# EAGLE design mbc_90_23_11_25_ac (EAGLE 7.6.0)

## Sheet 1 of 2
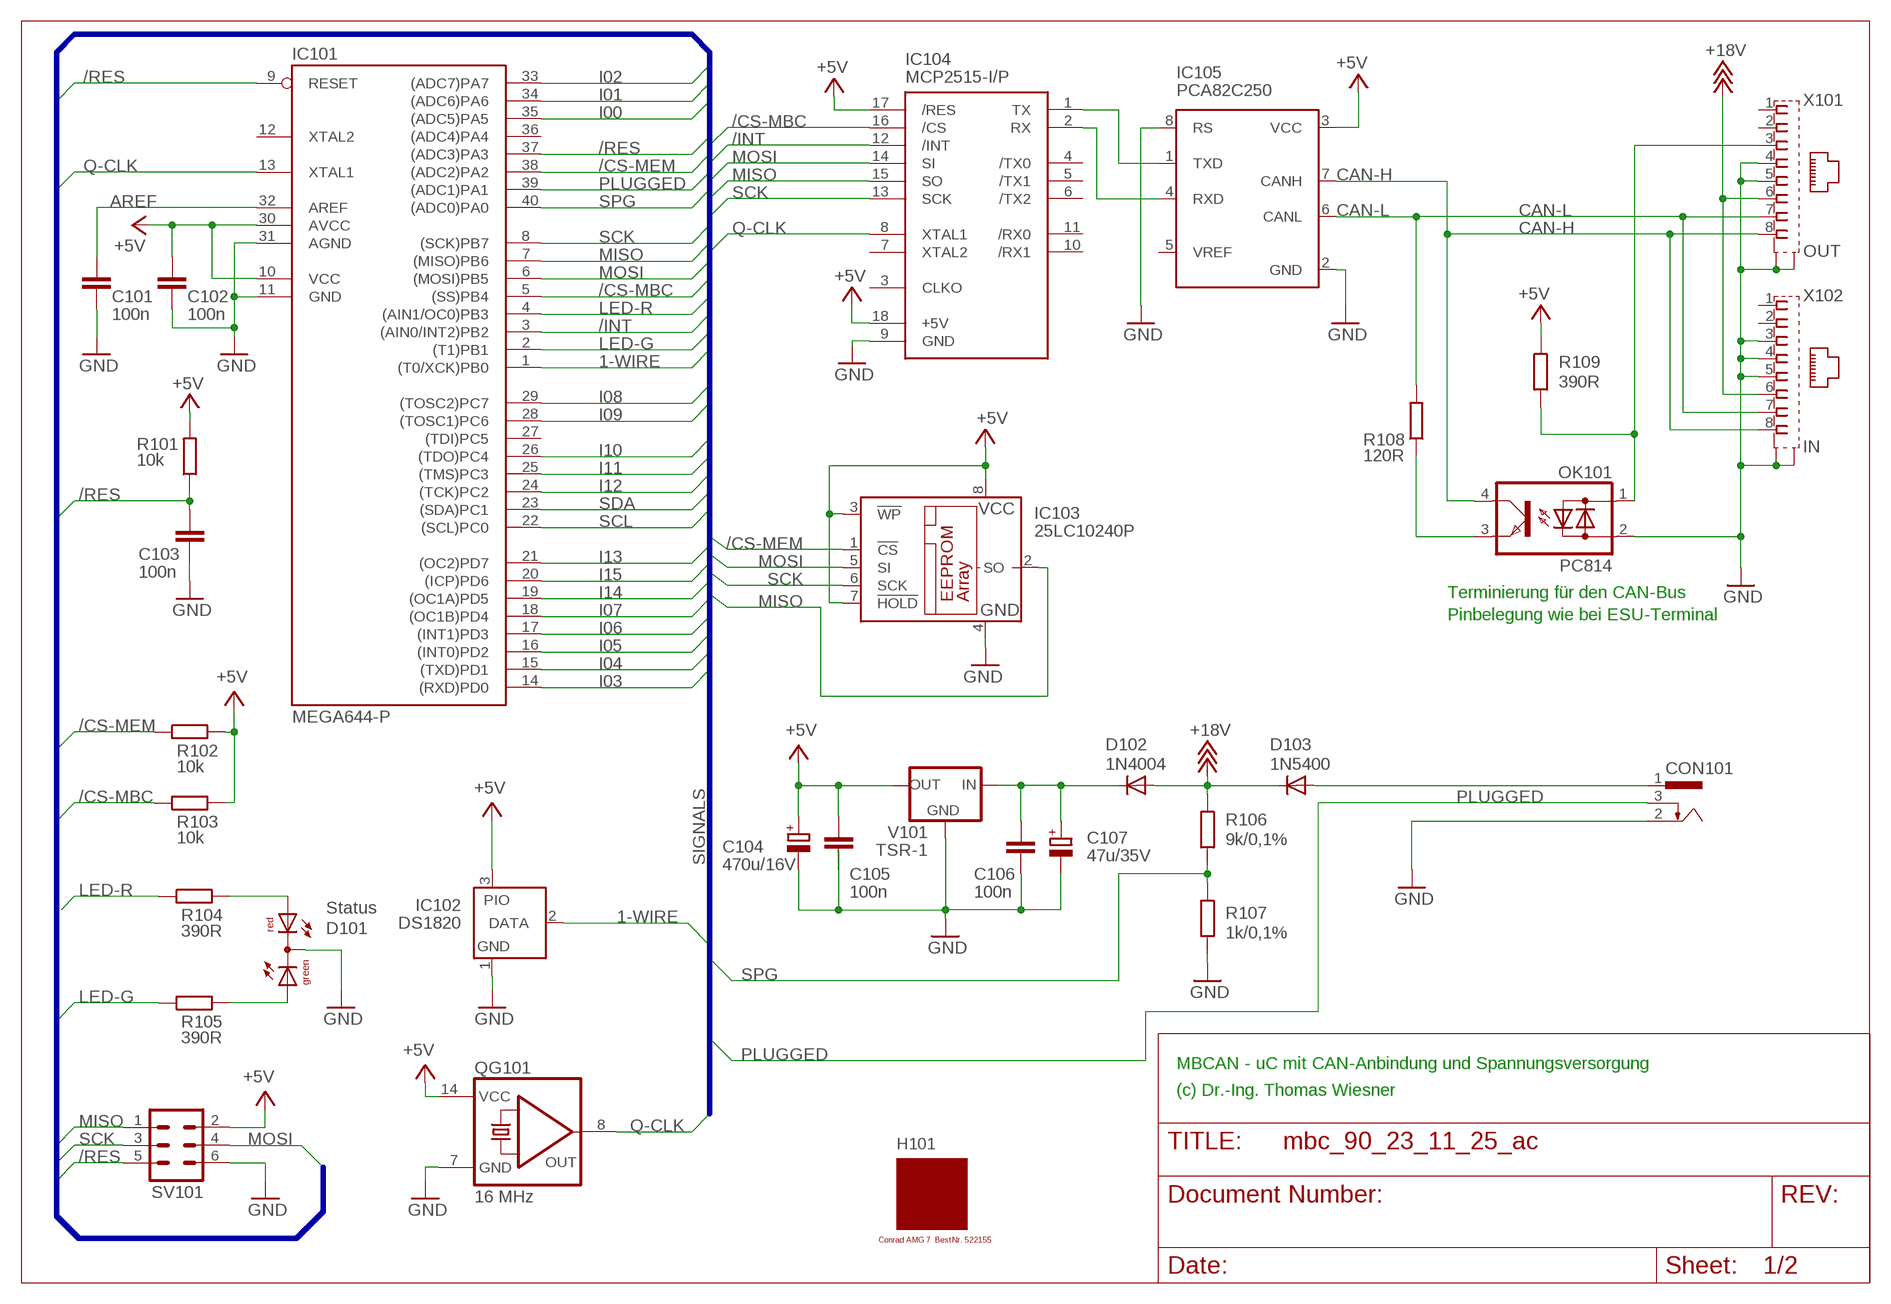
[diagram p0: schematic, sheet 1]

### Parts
C101  100n  C-EU025-025X050  [C025-025X050]
C102  100n  C-EU025-025X050  [C025-025X050]
C103  100n  C-EU025-025X050  [C025-025X050]
C104  470u/16V  CPOL-EUE3.5-8  [E3,5-8]
C105  100n  C-EU025-025X050  [C025-025X050]
C106  100n  C-EU025-025X050  [C025-025X050]
C107  47u/35V  CPOL-EUE2.5-7  [E2,5-7]
CON101  POWER-JACK  [POWER-JACK]
D101  Status  DUOLED5MM  [DUOLED5MM]
D102  1N4004  [DO41-10]
D103  1N5400  [DO201-15]
H101  MODULGEHÄUSE-AMG-7  [MODULGEHÄUSE-1]
IC101  MEGA644-P  MEGA323-P  [DIL40]
IC102  DS1820  DS2405  [TO92-]
IC103  25LC10240P  25LC040P  [DIL8]
IC104  MCP2515-I/P  MCP2510-I/P  [DIL18]
IC105  PCA82C250  [DIL08]
OK101  PC814  [DIL04]
QG101  16 MHz  QG5860  [DIL14S]
R101  10k  R-EU_0207/10  [0207/10]
R102  10k  R-EU_0207/10  [0207/10]
R103  10k  R-EU_0207/10  [0207/10]
R104  390R  R-EU_0207/10  [0207/10]
R105  390R  R-EU_0207/10  [0207/10]
R106  9k/0,1%  R-EU_0207/10  [0207/10]
R107  1k/0,1%  R-EU_0207/10  [0207/10]
R108  120R  R-EU_0207/10  [0207/10]
R109  390R  R-EU_0207/10  [0207/10]
SV101  ML6  [ML6]
V101  TSR-1  [TRACO-TSR-1]
X101  OUT  0446200002  [0446200002]
X102  IN  0446200002  [0446200002]

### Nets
1-WIRE: IC101.1((T0/XCK)PB0) IC102.2(DATA)
+5V: C102.1 C104.+ C105.1 IC101.10(VCC) IC101.30(AVCC) IC102.3(PIO) IC103.3(!WP) IC103.7(!HOLD) IC103.8(VCC) IC104.17(/RES) IC104.18(+5V) IC105.3(VCC) QG101.14(VCC) R101.2 R102.2 R103.2 R109.1 SV101.2 V101.OUT ; also sheet 2
+18V: D102.A D103.C R106.1 X101.6 X102.6
/CS-MBC: IC101.5((SS)PB4) IC104.16(/CS) R103.1
/CS-MEM: IC101.38((ADC2)PA2) IC103.1(!CS) R102.1
/INT: IC101.3((AIN0/INT2)PB2) IC104.12(/INT)
/RES: C103.1 IC101.9(RESET) IC101.37((ADC3)PA3) R101.1 SV101.5
AREF: C101.1 IC101.32(AREF)
CAN-H: IC105.7(CANH) OK101.4(C) X101.8 X102.8
CAN-L: IC105.6(CANL) R108.2 X101.7 X102.7
GND: C101.2 C102.2 C103.2 C104.- C105.2 C106.2 C107.- CON101.2 D101.K(C) IC101.11(GND) IC101.31(AGND) IC102.1(GND) IC103.4(GND) IC104.9(GND) IC105.2(GND) IC105.8(RS) QG101.7(GND) R107.2 SV101.6 V101.GND X101.4 X101.5 X101.S@1(S1) X101.S@2(S2) X102.3 X102.4 X102.5 X102.S@1(S1) X102.S@2(S2) ; also sheet 2
I00: IC101.35((ADC5)PA5) ; also sheet 2
I01: IC101.34((ADC6)PA6) ; also sheet 2
I02: IC101.33((ADC7)PA7) ; also sheet 2
I03: IC101.14((RXD)PD0) ; also sheet 2
I04: IC101.15((TXD)PD1) ; also sheet 2
I05: IC101.16((INT0)PD2) ; also sheet 2
I06: IC101.17((INT1)PD3) ; also sheet 2
I07: IC101.18((OC1B)PD4) ; also sheet 2
I08: IC101.29((TOSC2)PC7) ; also sheet 2
I09: IC101.28((TOSC1)PC6) ; also sheet 2
I10: IC101.26((TDO)PC4) ; also sheet 2
I11: IC101.25((TMS)PC3) ; also sheet 2
I12: IC101.24((TCK)PC2) ; also sheet 2
I13: IC101.21((OC2)PD7) ; also sheet 2
I14: IC101.19((OC1A)PD5) ; also sheet 2
I15: IC101.20((ICP)PD6) ; also sheet 2
LED-G: IC101.2((T1)PB1) R105.1
LED-R: IC101.4((AIN1/OC0)PB3) R104.1
MISO: IC101.7((MISO)PB6) IC103.2(SO) IC104.15(SO) SV101.1
MOSI: IC101.6((MOSI)PB5) IC103.5(SI) IC104.14(SI) SV101.4
N$1: IC104.1(TX) IC105.1(TXD)
N$2: IC104.2(RX) IC105.4(RXD)
N$4: OK101.3(E) R108.1
N$6: C106.1 C107.+ D102.C V101.IN
N$7: OK101.1(AC1) R109.2 X101.3
N$9: D101.AR R104.2
N$13: D101.AG R105.2
PLUGGED: CON101.3 IC101.39((ADC1)PA1)
Q-CLK: IC101.13(XTAL1) IC104.8(XTAL1) QG101.8(OUT)
SCK: IC101.8((SCK)PB7) IC103.6(SCK) IC104.13(SCK) SV101.3
SCL: IC101.22((SCL)PC0) ; also sheet 2
SDA: IC101.23((SDA)PC1) ; also sheet 2
SPG: IC101.40((ADC0)PA0) R106.2 R107.1
V-NETZTEIL1: CON101.1 D103.A
Unconnected: IC101.12(XTAL2) IC101.27((TDI)PC5) IC101.36((ADC4)PA4) IC104.3(CLKO) IC104.4(/TX0) IC104.5(/TX1) IC104.6(/TX2) IC104.7(XTAL2) IC104.10(/RX1) IC104.11(/RX0) IC105.5(VREF) OK101.2(AC2) X101.1 X101.2 X102.1 X102.2

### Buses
SIGNALS

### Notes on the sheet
- Terminierung für den CAN-Bus
- Pinbelegung wie bei ESU-Terminal
- MBCAN - uC mit CAN-Anbindung und Spannungsversorgung
- (c) Dr.-Ing. Thomas Wiesner

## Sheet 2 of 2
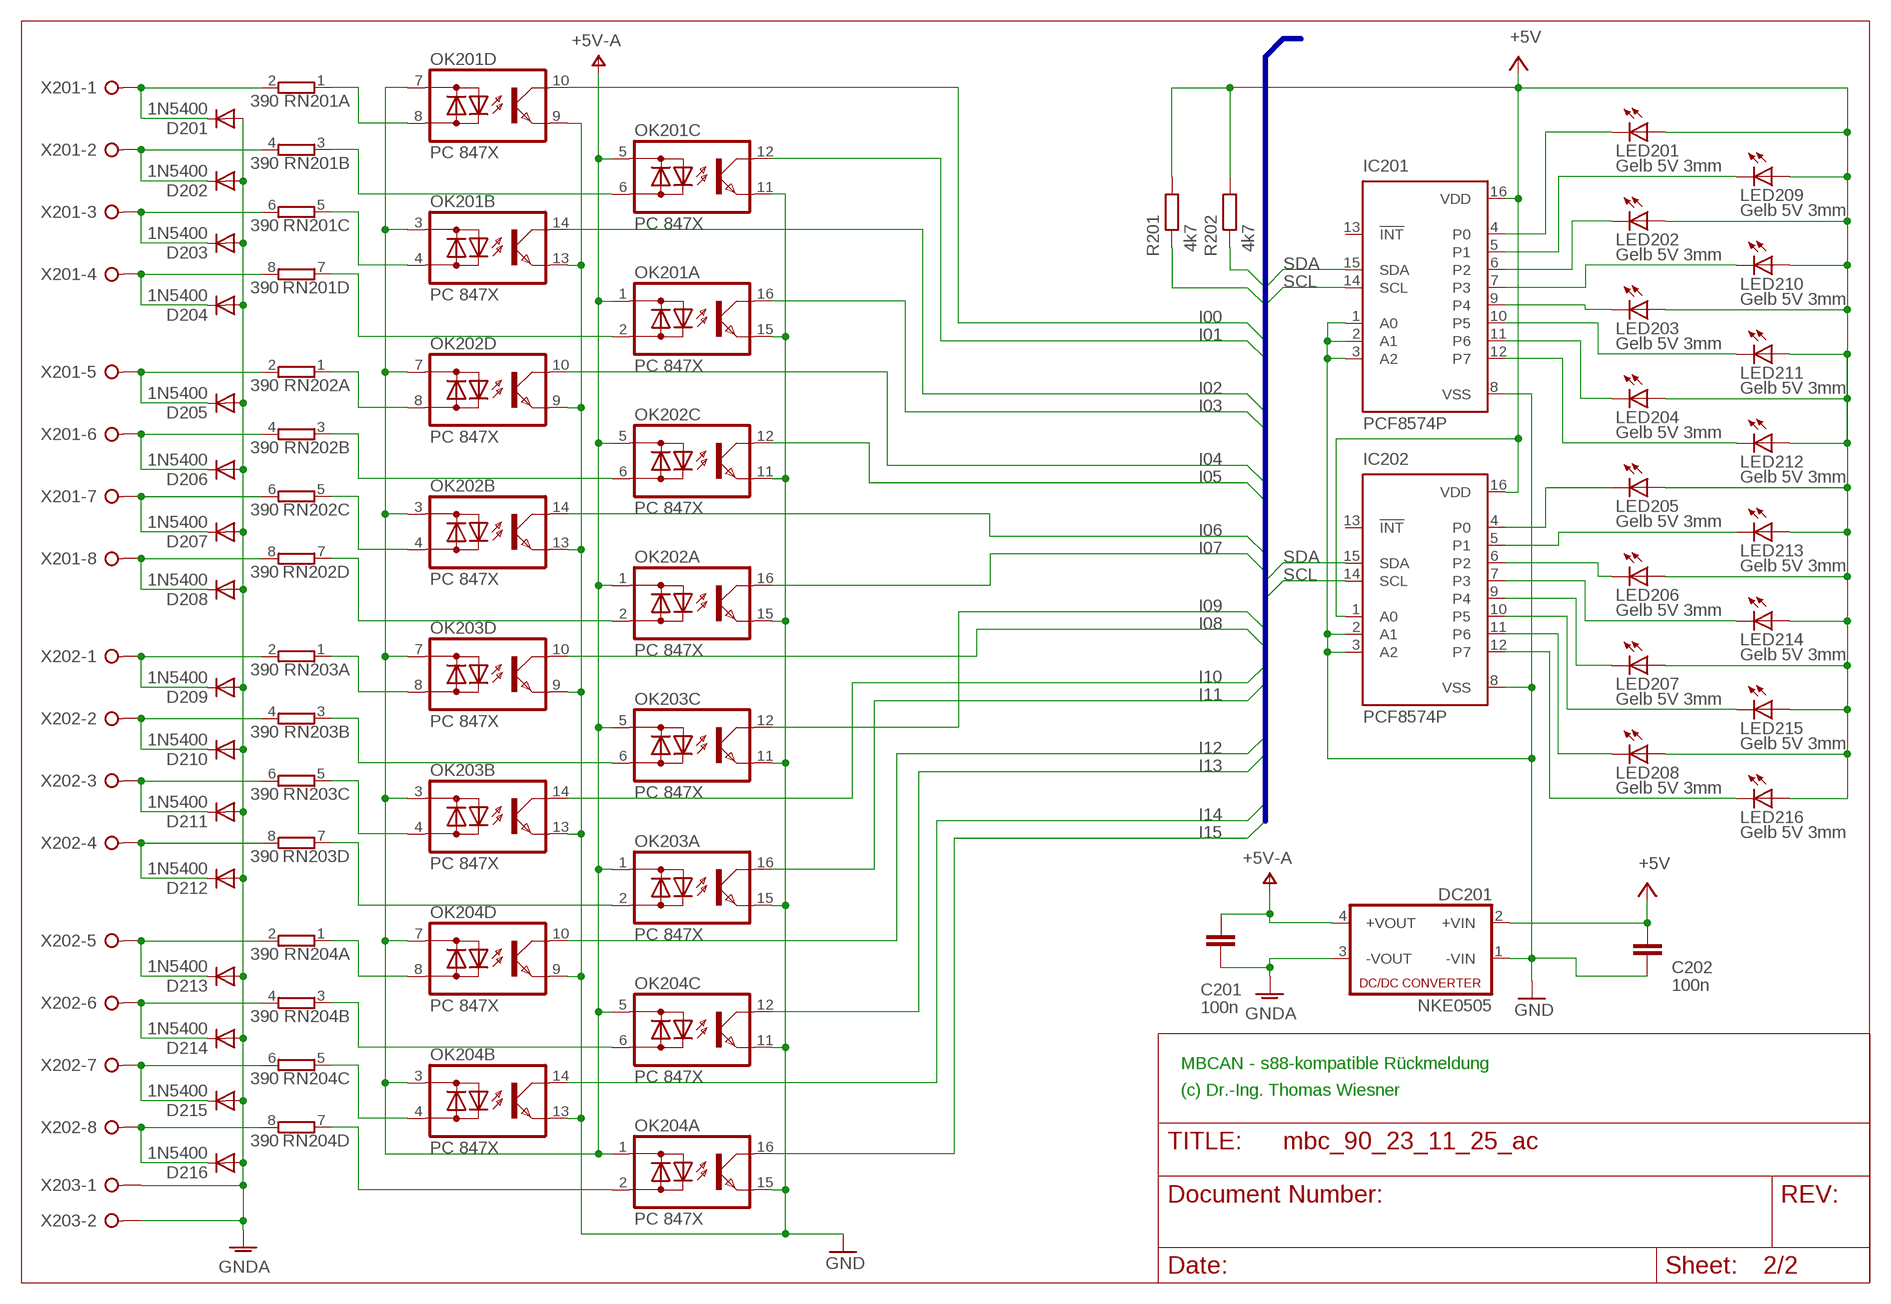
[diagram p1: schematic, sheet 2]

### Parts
C201  100n  C-EU025-025X050  [C025-025X050]
C202  100n  C-EU025-025X050  [C025-025X050]
D201  1N5400  [DO201-15]
D202  1N5400  [DO201-15]
D203  1N5400  [DO201-15]
D204  1N5400  [DO201-15]
D205  1N5400  [DO201-15]
D206  1N5400  [DO201-15]
D207  1N5400  [DO201-15]
D208  1N5400  [DO201-15]
D209  1N5400  [DO201-15]
D210  1N5400  [DO201-15]
D211  1N5400  [DO201-15]
D212  1N5400  [DO201-15]
D213  1N5400  [DO201-15]
D214  1N5400  [DO201-15]
D215  1N5400  [DO201-15]
D216  1N5400  [DO201-15]
DC201  NKE0505  NME  [NME]
IC201  PCF8574P  [DIL16]
IC202  PCF8574P  [DIL16]
LED201  Gelb 5V 3mm  LED3MM  [LED3MM]
LED202  Gelb 5V 3mm  LED3MM  [LED3MM]
LED203  Gelb 5V 3mm  LED3MM  [LED3MM]
LED204  Gelb 5V 3mm  LED3MM  [LED3MM]
LED205  Gelb 5V 3mm  LED3MM  [LED3MM]
LED206  Gelb 5V 3mm  LED3MM  [LED3MM]
LED207  Gelb 5V 3mm  LED3MM  [LED3MM]
LED208  Gelb 5V 3mm  LED3MM  [LED3MM]
LED209  Gelb 5V 3mm  LED3MM  [LED3MM]
LED210  Gelb 5V 3mm  LED3MM  [LED3MM]
LED211  Gelb 5V 3mm  LED3MM  [LED3MM]
LED212  Gelb 5V 3mm  LED3MM  [LED3MM]
LED213  Gelb 5V 3mm  LED3MM  [LED3MM]
LED214  Gelb 5V 3mm  LED3MM  [LED3MM]
LED215  Gelb 5V 3mm  LED3MM  [LED3MM]
LED216  Gelb 5V 3mm  LED3MM  [LED3MM]
OK201  PC 847X  TIL196  [DIL16]
OK202  PC 847X  TIL196  [DIL16]
OK203  PC 847X  TIL196  [DIL16]
OK204  PC 847X  TIL196  [DIL16]
R201  4k7  R-EU_0207/10  [0207/10]
R202  4k7  R-EU_0207/10  [0207/10]
RN201  390  E4R  [SIL8]
RN202  390  E4R  [SIL8]
RN203  390  E4R  [SIL8]
RN204  390  E4R  [SIL8]
X201  W237-08P  [W237-8P]
X202  W237-08P  [W237-8P]
X203  W237-02P  [W237-132]

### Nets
+5V: C202.1 DC201.2(+VIN) IC201.16(VDD) IC202.1(A0) IC202.16(VDD) LED201.A LED202.A LED203.A LED204.A LED205.A LED206.A LED207.A LED208.A LED209.A LED210.A LED211.A LED212.A LED213.A LED214.A LED215.A LED216.A R201.2 R202.2 ; also sheet 1
GND: C202.2 DC201.1(-VIN) IC201.1(A0) IC201.2(A1) IC201.3(A2) IC201.8(VSS) IC202.2(A1) IC202.3(A2) IC202.8(VSS) OK201.9(D:E) OK201.11(C:E) OK201.13(B:E) OK201.15(A:E) OK202.9(D:E) OK202.11(C:E) OK202.13(B:E) OK202.15(A:E) OK203.9(D:E) OK203.11(C:E) OK203.13(B:E) OK203.15(A:E) OK204.9(D:E) OK204.11(C:E) OK204.13(B:E) OK204.15(A:E) ; also sheet 1
GNDA: C201.2 D201.A D202.A D203.A D204.A D205.A D206.A D207.A D208.A D209.A D210.A D211.A D212.A D213.A D214.A D215.A D216.A DC201.3(-VOUT) X203.1 X203.2
I00: OK201.10(D:C) ; also sheet 1
I01: OK201.12(C:C) ; also sheet 1
I02: OK201.14(B:C) ; also sheet 1
I03: OK201.16(A:C) ; also sheet 1
I04: OK202.10(D:C) ; also sheet 1
I05: OK202.12(C:C) ; also sheet 1
I06: OK202.14(B:C) ; also sheet 1
I07: OK202.16(A:C) ; also sheet 1
I08: OK203.10(D:C) ; also sheet 1
I09: OK203.12(C:C) ; also sheet 1
I10: OK203.14(B:C) ; also sheet 1
I11: OK203.16(A:C) ; also sheet 1
I12: OK204.10(D:C) ; also sheet 1
I13: OK204.12(C:C) ; also sheet 1
I14: OK204.14(B:C) ; also sheet 1
I15: OK204.16(A:C) ; also sheet 1
N$15: IC201.9(P4) LED203.K(C)
N$16: D215.C RN204.6 X202.7
N$17: D216.C RN204.8 X202.8
N$18: D213.C RN204.2 X202.5
N$19: D214.C RN204.4 X202.6
N$20: D211.C RN203.6 X202.3
N$21: D212.C RN203.8 X202.4
N$22: D209.C RN203.2 X202.1
N$23: D210.C RN203.4 X202.2
N$24: D207.C RN202.6 X201.7
N$25: D208.C RN202.8 X201.8
N$26: D205.C RN202.2 X201.5
N$27: D206.C RN202.4 X201.6
N$28: D203.C RN201.6 X201.3
N$29: D204.C RN201.8 X201.4
N$30: D201.C RN201.2 X201.1
N$31: IC201.10(P5) LED211.K(C)
N$32: OK204.2(A:AC2) RN204.7
N$35: OK204.4(B:AC2) RN204.5
N$36: OK204.6(C:AC2) RN204.3
N$37: OK204.8(D:AC2) RN204.1
N$38: OK203.2(A:AC2) RN203.7
N$39: OK203.4(B:AC2) RN203.5
N$40: OK203.6(C:AC2) RN203.3
N$41: OK203.8(D:AC2) RN203.1
N$42: OK202.2(A:AC2) RN202.7
N$43: OK202.4(B:AC2) RN202.5
N$44: OK202.6(C:AC2) RN202.3
N$45: OK202.8(D:AC2) RN202.1
N$46: OK201.2(A:AC2) RN201.7
N$47: D202.C RN201.4 X201.2
N$48: OK201.4(B:AC2) RN201.5
N$49: IC202.4(P0) LED205.K(C)
N$50: IC201.4(P0) LED201.K(C)
N$51: IC201.5(P1) LED209.K(C)
N$52: IC201.6(P2) LED202.K(C)
N$53: IC201.7(P3) LED210.K(C)
N$54: IC201.11(P6) LED204.K(C)
N$55: IC201.12(P7) LED212.K(C)
N$56: IC202.9(P4) LED207.K(C)
N$57: IC202.5(P1) LED213.K(C)
N$58: IC202.6(P2) LED206.K(C)
N$59: IC202.7(P3) LED214.K(C)
N$60: IC202.10(P5) LED215.K(C)
N$61: IC202.11(P6) LED208.K(C)
N$62: IC202.12(P7) LED216.K(C)
N$64: OK201.6(C:AC2) RN201.3
N$65: OK201.8(D:AC2) RN201.1
SCL: IC201.14(SCL) IC202.14(SCL) R201.1 ; also sheet 1
SDA: IC201.15(SDA) IC202.15(SDA) R202.1 ; also sheet 1
V+: C201.1 DC201.4(+VOUT) OK201.1(A:AC1) OK201.3(B:AC1) OK201.5(C:AC1) OK201.7(D:AC1) OK202.1(A:AC1) OK202.3(B:AC1) OK202.5(C:AC1) OK202.7(D:AC1) OK203.1(A:AC1) OK203.3(B:AC1) OK203.5(C:AC1) OK203.7(D:AC1) OK204.1(A:AC1) OK204.3(B:AC1) OK204.5(C:AC1) OK204.7(D:AC1) ; supply symbol labelled +5V-A
Unconnected: IC201.13(!INT) IC202.13(!INT)

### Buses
B$1

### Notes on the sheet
- MBCAN - s88-kompatible Rückmeldung
- (c) Dr.-Ing. Thomas Wiesner

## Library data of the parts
C101-C103 C105 C106 C201 C202 = rcl:C-EU: CAPACITOR, European symbol
C104 C107 = rcl:CPOL-EU: POLARIZED CAPACITOR, European symbol
CON101 = mbc:POWER-JACK: Power-Stecker für 2,5 mm Hohlbuchse
D101 = led:DUOLED5MM: DUO LED 2 colors, 5 mm, round
D102 = diode:1N4004: DIODE
D103 D201-D216 = diode:1N5400: DIODE
DC201 = dc-dc-converter:NME: DC-DC CONVERTER; MF: C & D TECHNOLOGIES, INC; MPN: NME1205D; OC_FARNELL: 1021466; OC_NEWARK: 98B8198
H101 = mbc:MODULGEHÄUSE-AMG-7: Gehäuse
IC101 = atmel:MEGA323-P: MICROCONTROLLER 32 Kbytes FLASH 2 Kbytes SRAM 1 Kbytes EEPROM USART 8-channel 10 bit ADC Source: avr.lbr; OC_FARNELL: unknown; OC_NEWARK: unknown
IC102 = maxim:DS2405: Addressable Switch DALLAS Semiconductor; MF: DALLAS SEMICONDUCTOR; MPN: DS2405; OC_FARNELL: 1188025; OC_NEWARK: 06F4645
IC103 = microchip:25*: Serial EEPROM 4K/ 8K , SPI bus; MF: MICROCHIP; MPN: 25LC040/P; OC_FARNELL: 9758100; OC_NEWARK: 96K4091
IC104 = mbc:MCP2510: BASIC-CAN 2.0a Controller Stand-alone CAN controller von Microchip
IC105 = micro-philips:PCA82C250: CAN CONTROLLER INTERFACE; OC_FARNELL: 3692358; OC_NEWARK: unknown
IC201 IC202 = micro-philips:PCF8574: I2C-Bus Remote 8-bit I/O expander http://www.semiconductors.philips.com/acrobat_download/datasheets/PCF8574_4.pdf; MPN: PCF8574PN; OC_FARNELL: 204020; OC_NEWARK: 11N8515
LED201-LED216 = led:LED: LED
OK101 = optocoupler:PC814: SHARP OPTO COUPLER; OC_FARNELL: 9707662; OC_NEWARK: unknown
OK201-OK204 = optocoupler:TIL196: TEXAS INSTRUMENTS OPTO COUPLER; MPN: TIL 196; OC_FARNELL: 1683367; OC_NEWARK: 05R6476
QG101 = crystal:QG5860: CRYSTAL RESONATOR; OC_FARNELL: unknown; OC_NEWARK: unknown
R101-R109 R201 R202 = resistor:R-EU_: RESISTOR, European symbol
RN201-RN204 = resistor-sil:E4R: SIL RESISTOR; OC_FARNELL: unknown; OC_NEWARK: unknown
SV101 = con-ml:ML6: HARTING; OC_FARNELL: unknown; OC_NEWARK: unknown
V101 = mbc:TSR-1: Spannungsregler Hersteller: TRACO Typ: TSR-1 5V: TSR 1-2450 Spg: 5V Strom: 1A Reichelt TSR 1-2450
X101 X102 = mbc:0446200002: RJ-45 INVERTED MODULAR JACK ASSEMBLY WITH RJ-11 KEEPOUT FEATURE Source: Data sheet MOLEX 0446200002 BUCHSE, RJ45, GESCHIRMT Source: Farnell; MF: MOLEX; MPN: 0446200002; OC_FARNELL: 9251910
X201 X202 = con-wago-508:W237-08P: WAGO SREW CLAMP; OC_FARNELL: unknown; OC_NEWARK: unknown
X203 = con-wago-508:W237-02P: WAGO SREW CLAMP; OC_FARNELL: unknown; OC_NEWARK: unknown

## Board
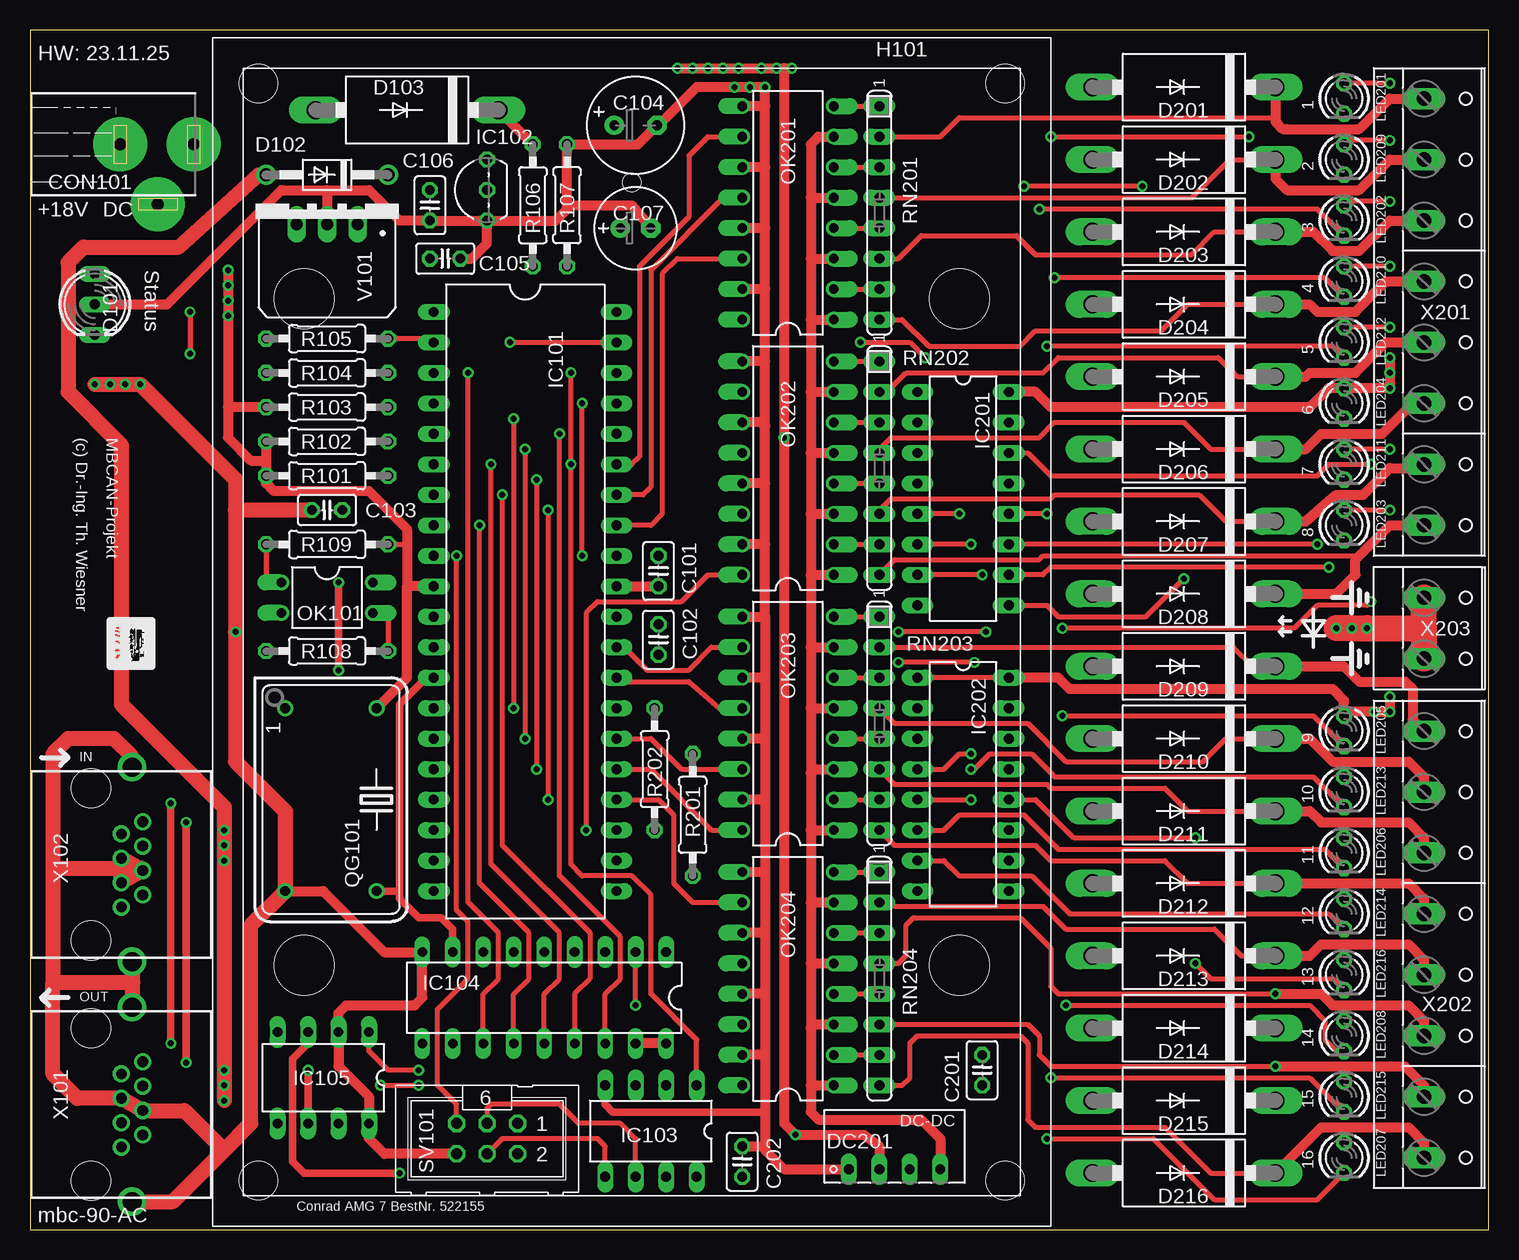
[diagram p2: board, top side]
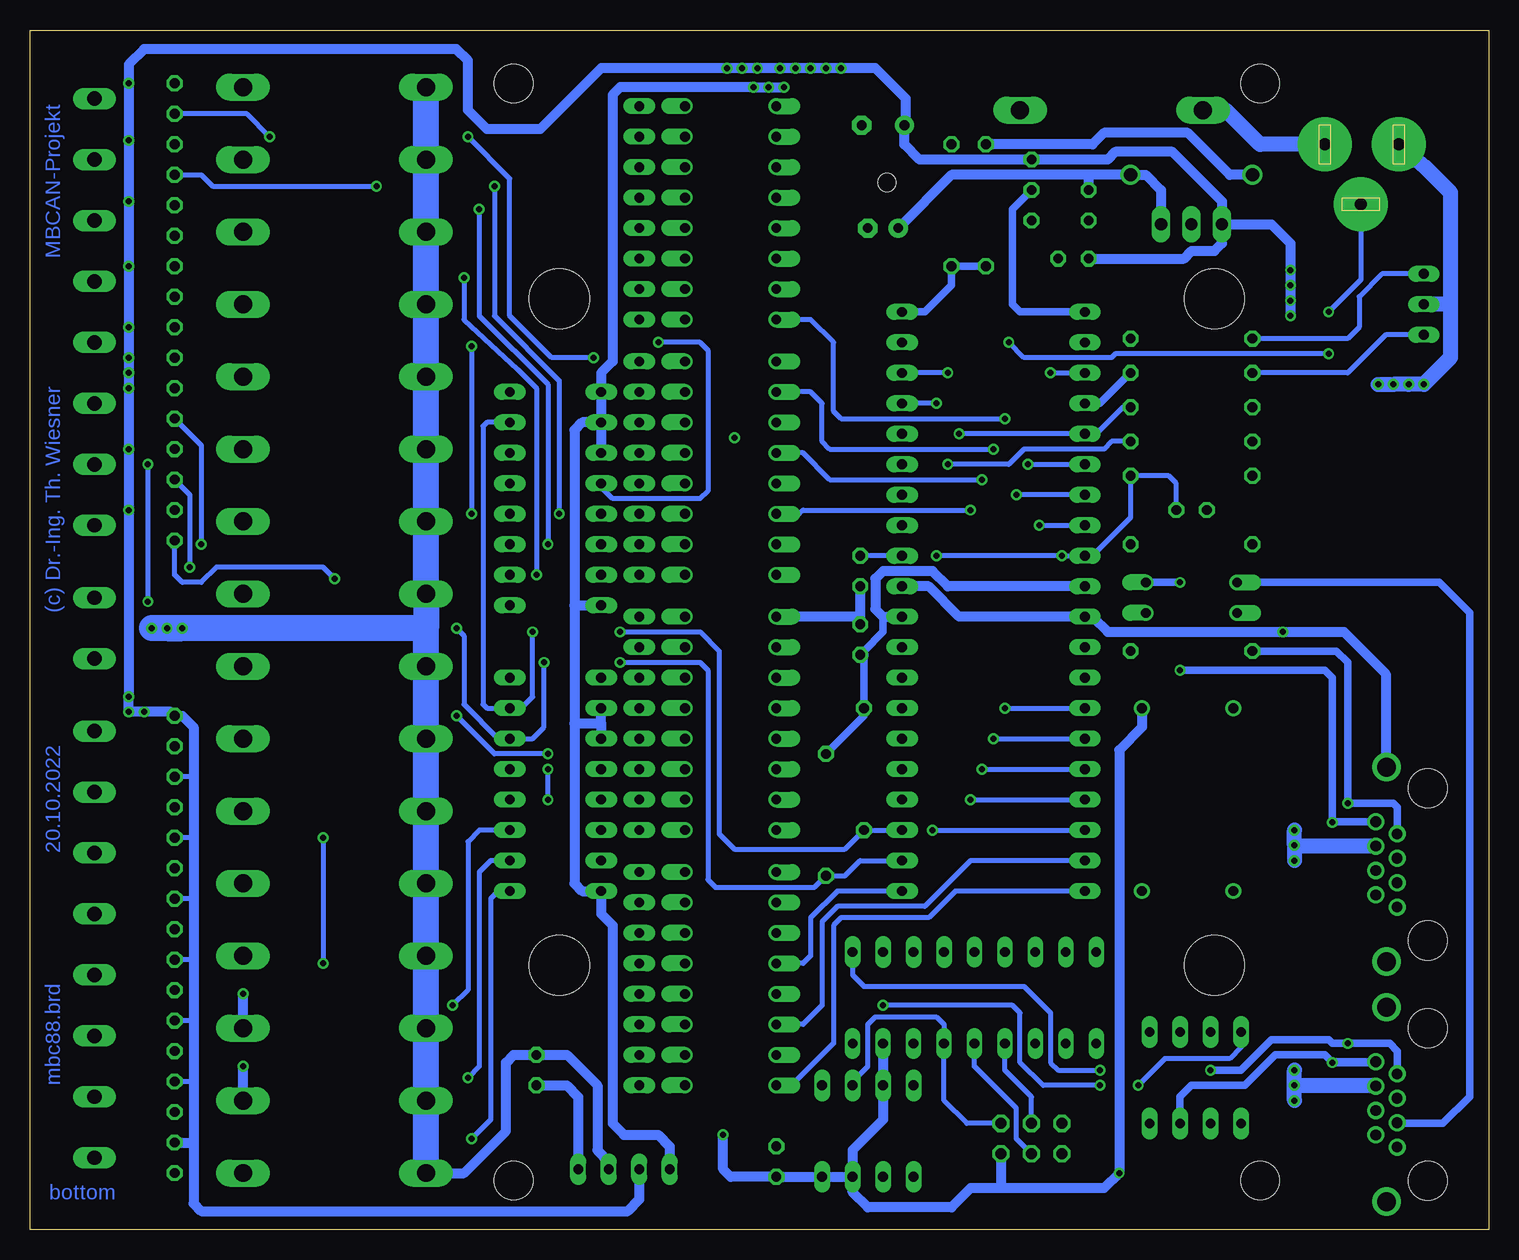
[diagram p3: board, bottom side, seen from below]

Size 121.59 x 99.99 mm. Coordinates in mm from the lower left corner, seen from the top.
Outline: 0,99.99 0,0 121.59,0 121.59,99.99 0,99.99
Copper layers (1*16): Top 0.035mm / dielectric 1.5mm / Bottom 0.035mm
Design rules "default *": minimum track width 10mil, minimum drill 0.5mm, track to track 8mil, track to pad 8mil, pad to pad 8mil, via to via 8mil, smd to smd 8mil, copper to edge 40mil, drill to drill 8mil, minimum pad ring 10mil, minimum via ring 8mil, stop-mask expansion 4mil, vias tented up to drill 0mil, thermal gap 10mil

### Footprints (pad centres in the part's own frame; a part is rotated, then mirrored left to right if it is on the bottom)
C025-025X050 = drill 0.813 octagon: 1 -1.27,0; 2 1.27,0
E3,5-8 = drill 0.813 pad 1.6: + -1.778,0 | drill 0.813 pad 1.6 octagon: - 1.778,0
E2,5-7 = drill 0.813 pad 1.6: + -1.27,0 | drill 0.813 pad 1.6 octagon: - 1.27,0
POWER-JACK = drill 1 pad 4.5: 1 0,6.03; 2 0,-0.12; 3 5,3.03
DUOLED5MM = drill 0.813 long: AG -2.54,0; AR 2.54,0; K 0,0
DO41-10 = drill 1.118: A 5.08,0; C -5.08,0
DO201-15 = drill 1.499 long: A 7.62,0; C -7.62,0
NME = drill 0.813 long: 1 0,3.81; 2 0,1.27; 3 0,-1.27; 4 0,-3.81
MODULGEHÄUSE-1 = hole 3.2: -45.72,-31.115; -45.72,31.115; 45.72,31.115; 45.72,-31.115 | hole 5: -27.781,-27.305; 27.781,-27.305; -27.781,27.305; 27.781,27.305 | hole 1.5: -37.465,0
DIL40 = drill 0.813 long: 1 -24.13,-7.62; 2 -21.59,-7.62; 3 -19.05,-7.62; 4 -16.51,-7.62; 5 -13.97,-7.62; 6 -11.43,-7.62; 7 -8.89,-7.62; 8 -6.35,-7.62; 9 -3.81,-7.62; 10 -1.27,-7.62; 11 1.27,-7.62; 12 3.81,-7.62; 13 6.35,-7.62; 14 8.89,-7.62; 15 11.43,-7.62; 16 13.97,-7.62; 17 16.51,-7.62; 18 19.05,-7.62; 19 21.59,-7.62; 20 24.13,-7.62; 21 24.13,7.62; 22 21.59,7.62; 23 19.05,7.62; 24 16.51,7.62; 25 13.97,7.62; 26 11.43,7.62; 27 8.89,7.62; 28 6.35,7.62; 29 3.81,7.62; 30 1.27,7.62; 31 -1.27,7.62; 32 -3.81,7.62; 33 -6.35,7.62; 34 -8.89,7.62; 35 -11.43,7.62; 36 -13.97,7.62; 37 -16.51,7.62; 38 -19.05,7.62; 39 -21.59,7.62; 40 -24.13,7.62
TO92- = drill 0.813 octagon: 1 -2.54,0; 2 0,0; 3 2.54,0
DIL8 = drill 0.813 long: 1 -3.81,-3.81; 2 -1.27,-3.81; 3 1.27,-3.81; 4 3.81,-3.81; 5 3.81,3.81; 6 1.27,3.81; 7 -1.27,3.81; 8 -3.81,3.81
DIL18 = drill 0.813 long: 1 -10.16,-3.81; 2 -7.62,-3.81; 3 -5.08,-3.81; 4 -2.54,-3.81 | drill 0.8 long: 5 0,-3.81; 6 2.54,-3.81; 7 5.08,-3.81; 8 7.62,-3.81; 9 10.16,-3.81; 10 10.16,3.81; 11 7.62,3.81; 12 5.08,3.81; 13 2.54,3.81; 14 0,3.81; 15 -2.54,3.81; 16 -5.08,3.81; 17 -7.62,3.81; 18 -10.16,3.81
DIL08 = drill 0.813 long: 1 -3.81,-3.81; 2 -1.27,-3.81; 3 1.27,-3.81; 4 3.81,-3.81; 5 3.81,3.81; 6 1.27,3.81; 7 -1.27,3.81; 8 -3.81,3.81
DIL16 = drill 0.813 long: 1 -8.89,-3.81; 2 -6.35,-3.81; 3 -3.81,-3.81; 4 -1.27,-3.81; 5 1.27,-3.81; 6 3.81,-3.81; 7 6.35,-3.81; 8 8.89,-3.81; 9 8.89,3.81; 10 6.35,3.81; 11 3.81,3.81; 12 1.27,3.81; 13 -1.27,3.81; 14 -3.81,3.81; 15 -6.35,3.81; 16 -8.89,3.81
LED3MM = drill 0.813 octagon: A -1.27,0; K 1.27,0
DIL04 = drill 0.813 offset: 1 -1.27,-3.81; 2 1.27,-3.81; 3 1.27,3.81; 4 -1.27,3.81
DIL16' = drill 0.813 offset: 1 -8.89,-3.81; 2 -6.35,-3.81; 3 -3.81,-3.81; 4 -1.27,-3.81; 5 1.27,-3.81; 6 3.81,-3.81; 7 6.35,-3.81; 8 8.89,-3.81; 9 8.89,3.81; 10 6.35,3.81; 11 3.81,3.81; 12 1.27,3.81; 13 -1.27,3.81; 14 -3.81,3.81; 15 -6.35,3.81; 16 -8.89,3.81
DIL14S = drill 0.813: 1 -7.62,-3.81; 7 7.62,-3.81; 8 7.62,3.81; 14 -7.62,3.81
0207/10 = drill 0.813 octagon: 1 -5.08,0; 2 5.08,0
SIL8 = drill 0.813 long: 1 -8.89,0; 2 -6.35,0; 3 -3.81,0; 4 -1.27,0; 5 1.27,0; 6 3.81,0; 7 6.35,0; 8 8.89,0
ML6 = drill 0.914 octagon: 1 -2.54,-1.27; 2 -2.54,1.27; 3 0,-1.27; 4 0,1.27; 5 2.54,-1.27; 6 2.54,1.27
TRACO-TSR-1 = drill 1.016 long: GND 0,2.54; IN -2.54,2.54; OUT 2.54,2.54
0446200002 = drill 0.889 pad 1.422: 1 3.556,2.54; 2 2.54,4.318; 3 1.524,2.54; 4 0.508,4.318; 5 -0.508,2.54; 6 -1.524,4.318; 7 -2.54,2.54; 8 -3.556,4.318 | drill 1.575 pad 2.286: S@1 -8.103,3.429; S@2 8.103,3.429 | hole 3.251: 6.35,0; -6.35,0
W237-8P = drill 1.194 long: 1 -17.78,-0.635; 2 -12.7,-0.635; 3 -7.62,-0.635; 4 -2.54,-0.635; 5 2.54,-0.635; 6 7.62,-0.635; 7 12.7,-0.635; 8 17.78,-0.635
W237-132 = drill 1.194 long: 1 -2.54,-0.635; 2 2.54,-0.635

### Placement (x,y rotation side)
C101  52.39,54.91 270 top
C102  52.39,49.19 90 top
C103  24.77,59.99 180 top
C104  50.48,92.06 0 top
C105  34.61,80.94 0 top
C106  33.34,85.39 270 top
C107  50.48,83.48 0 top
C201  79.38,13.32 90 top
C202  59.37,5.7 90 top
CON101  7.62,90.47 270 top
D101  5.4,77.13 270 top
D102  24.77,87.93 180 top
D103  31.43,93.33 180 top
D201  96.2,95.23 180 top
D202  96.2,89.2 180 top
D203  96.2,83.17 180 top
D204  96.2,77.13 180 top
D205  96.2,71.1 180 top
D206  96.2,65.07 180 top
D207  96.2,59.03 180 top
D208  96.2,53 180 top
D209  96.2,46.97 180 top
D210  96.2,40.94 180 top
D211  96.2,34.9 180 top
D212  96.2,28.87 180 top
D213  96.2,22.84 180 top
D214  96.2,16.81 180 top
D215  96.2,10.78 180 top
D216  96.2,4.74 180 top
DC201  72.07,5.06 90 top
H101  50.16,49.83 270 top
IC101  41.27,52.37 270 top
IC102  38.1,86.66 90 top
IC103  51.75,8.24 180 top
IC104  42.86,19.35 180 top
IC105  24.45,12.68 180 top
IC201  77.79,60.94 270 top
IC202  77.79,37.13 270 top
LED201  109.54,94.28 270 top
LED202  109.54,84.12 270 top
LED203  109.54,58.72 270 top
LED204  109.54,68.88 270 top
LED205  109.54,41.57 270 top
LED206  109.54,31.41 270 top
LED207  109.54,6.01 270 top
LED208  109.54,16.17 270 top
LED209  109.54,89.2 270 top
LED210  109.54,79.04 270 top
LED211  109.54,63.8 270 top
LED212  109.54,73.96 270 top
LED213  109.54,36.49 270 top
LED214  109.54,26.33 270 top
LED215  109.54,11.09 270 top
LED216  109.54,21.25 270 top
OK101  24.77,52.68 270 top
OK201  PC 847X  [DIL16']  63.18,84.75 90 top
OK202  PC 847X  [DIL16']  63.18,63.48 90 top
OK203  PC 847X  [DIL16']  63.18,42.21 90 top
OK204  PC 847X  [DIL16']  63.18,20.93 90 top
QG101  25.08,35.86 270 top
R101  24.77,62.84 180 top
R102  24.77,65.7 180 top
R103  24.77,68.56 180 top
R104  24.77,71.42 180 top
R105  24.77,74.28 180 top
R106  41.91,85.39 270 top
R107  44.77,85.39 90 top
R108  24.77,48.24 180 top
R109  24.77,57.13 180 top
R201  55.24,34.59 90 top
R202  52.07,38.4 90 top
RN201  70.8,84.75 270 top
RN202  70.8,63.48 270 top
RN203  70.8,42.21 270 top
RN204  70.8,20.93 270 top
SV101  38.1,7.6 180 top
V101  24.77,86.34 180 top
X101  5.08,10.46 270 top
X102  5.08,30.46 270 top
X201  116.84,76.5 270 top
X202  116.84,23.79 270 top
X203  116.84,50.14 270 top

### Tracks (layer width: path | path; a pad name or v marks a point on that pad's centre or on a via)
1-WIRE
  Bottom 0.61: IC102.2 39.69,85.07 39.69,77.13 39.05,76.5 IC101.1
+5V  (via drill 0.5)
  Top 0.406: v113.35,95.55 LED201.A | LED209.A 109.54,90.79 v113.35,90.79 | LED202.A 109.54,85.7 v113.35,85.7 | v113.35,80.31 LED210.A | v113.35,65.07 LED211.A | v113.35,59.99 LED203.A | IC202.16 IC202.1 | v113.35,75.23 LED212.A | R109.1 31.43,57.13
  Top 0.61: IC105.3 23.18,15.54 21.91,14.27 21.91,5.7 22.86,4.74 v30.8,4.74
  Top 0.813: IC104.18 IC104.17 | 31.43,53.64 31.43,57.13 31.43,58.4 28.26,61.57 20.32,61.57 19.68,62.21 R101.2 19.68,64.12 | v16.51,79.99 v16.51,78.72 v16.51,77.45 v16.51,76.18 16.51,68.56 | 16.51,68.56 16.51,66.02 18.41,64.12 19.68,64.12 | IC101.10 31.43,53.64 | v53.98,96.82 v55.24,96.82 v56.52,96.82 v57.78,96.82 v59.05,96.82 v60.96,96.82 v62.23,96.82 62.87,96.82 | 62.87,96.82 v63.5,96.82 | IC202.16 85.72,46.02 86.68,45.06 108.58,45.06 109.54,44.11 LED205.A 109.54,43.16 v112.08,43.16 v113.35,43.16 v113.35,44.43 | v113.35,72.69 v113.35,71.42 v113.35,70.15 LED204.A 108.27,70.15 106.68,68.56 85.09,68.56 83.82,69.83 IC201.16 | 62.87,96.82 v62.87,66.02 62.87,8.87 v63.82,7.92 69.53,7.92 70.8,6.97 DC201.2 | QG101.14 31.43,46.02 31.43,53.64 | R103.2 16.51,68.56 | R102.2 19.68,64.12
  Bottom 0.406: 107.95,37.76 LED213.A | 107.95,32.68 LED206.A | 107.95,27.6 LED214.A | 107.95,22.52 LED216.A | 107.95,17.44 LED208.A | 107.95,12.36 LED215.A
  Bottom 0.61: 50.48,51.1 50.48,49.83 52.07,48.24 52.07,47.92 R202.2 52.07,42.84 R201.2
  Bottom 0.813: V101.OUT 18.1,83.8 16.51,82.21 v16.51,79.99 v16.51,78.72 v16.51,77.45 v16.51,76.18 | QG101.14 28.89,41.89 30.8,39.98 v30.8,4.74 32.07,3.47 40.64,3.47 | IC101.10 45.09,53.64 46.35,54.91 50.48,54.91 51.12,54.27 51.12,51.73 50.48,51.1 IC101.30 | V101.OUT 22.23,85.7 26.35,89.83 31.11,89.83 31.75,89.2 IC102.3 47.43,89.2 48.7,90.47 C104.+ | 107.95,7.28 107.95,12.36 107.95,17.44 107.95,22.52 107.95,27.6 107.95,32.68 107.95,37.76 107.95,41.89 108.9,42.84 LED205.A 109.86,43.16 v112.08,43.16 v113.35,43.16 v113.35,44.43 v113.35,59.99 v113.35,65.07 v113.35,70.15 v113.35,71.42 v113.35,72.69 v113.35,75.23 v113.35,80.31 v113.35,85.7 v113.35,90.79 v113.35,95.55 113.35,97.14 112.08,98.41 86.04,98.41 85.09,97.45 85.09,93.33 83.5,91.74 79.06,91.74 73.98,96.82 v63.5,96.82 v62.23,96.82 v60.96,96.82 v59.05,96.82 v57.78,96.82 v56.52,96.82 v55.24,96.82 v53.98,96.82 51.12,96.82 48.58,94.28 48.58,92.06 | v63.82,7.92 63.82,5.06 63.18,4.43 C202.1 IC103.8 IC103.7 | IC104.17 IC103.3 50.48,9.19 53.02,6.65 IC103.7 | 40.64,3.47 43.18,3.47 44.77,1.89 51.75,1.89 53.02,3.15 IC103.7 | SV101.2 40.64,3.47 | C105.1 25.4,80.94 24.77,81.58 22.86,81.58 22.23,82.21 V101.OUT | LED207.A 107.95,7.28 | 107.95,7.28 107.95,2.2 107.31,1.57 71.75,1.57 70.8,2.52 DC201.2 | C102.1 52.07,47.92
+18V  (via drill 0.5)
  Top 0.813: R106.1 D103.C
  Top 1.27: D102.A 19.05,87.93 12.38,81.9 4.45,81.9 3.17,80.62 3.17,69.83 7.62,65.39 7.62,43.79 16.19,35.22 v16.19,33.32 v16.19,32.05 v16.19,30.78 v16.19,13.32 v16.19,12.04 v16.19,10.78
  Bottom 0.813: R106.1 33.02,90.47 32.07,91.42 25.08,91.42 21.59,87.93 D102.A
  Bottom 1.27: v16.19,12.04 9.46,12.04 X101.6 | v16.19,10.78 v16.19,12.04 | v16.19,12.04 v16.19,13.32 | X102.6 16.13,31.98 v16.19,32.05 | v16.19,32.05 v16.19,33.32 | v16.19,32.05 v16.19,30.78
/CS-MBC  (via drill 0.5)
  Top 0.406: IC104.16 47.94,19.66 49.21,20.93 49.21,24.43 44.13,29.51 v44.13,66.34
  Bottom 0.406: R103.1 30.48,68.56 32.7,66.34 IC101.5 v44.13,66.34
/CS-MEM  (via drill 0.5)
  Top 0.406: IC103.1 55.56,15.86 51.75,19.66 51.75,27.92 50.16,29.51 46.04,29.51 45.09,30.46 v45.09,63.8 v45.09,71.42
  Bottom 0.406: v45.09,71.42 IC101.38 | R102.1 31.43,65.7 32.07,65.07 38.73,65.07 40.01,63.8 v45.09,63.8
/INT  (via drill 0.5)
  Top 0.406: IC104.12 37.78,19.66 39.05,20.93 39.05,24.75 36.51,27.29 v36.51,71.42
  Bottom 0.406: v36.51,71.42 IC101.3
/RES  (via drill 0.5)
  Top 0.406: SV101.5 35.56,10.46 33.97,12.04 33.97,18.39 36.51,20.93 36.51,25.7 35.56,26.65 v35.56,56.18 | v46.04,56.18 v46.04,68.88
  Bottom 0.406: C103.1 26.04,62.21 26.67,62.84 R101.1 29.84,59.35 33.02,56.18 IC101.9 v35.56,56.18 v46.04,56.18 | v46.04,68.88 IC101.37
AREF
  Bottom 0.406: IC101.32 C101.1
CAN-H  (via drill 0.5)
  Top 0.61: v13.02,13.95 v13.02,33.95 | v25.72,46.65 v25.72,53.95
  Bottom 0.61: IC105.7 25.72,11.09 24.77,12.04 20.32,12.04 17.78,14.59 13.65,14.59 13.08,14.01 X101.8 9.46,14.01 9.53,13.95 v13.02,13.95 | v13.02,33.95 13.02,34.02 | 13.02,34.02 X102.8 | 13.02,34.02 13.02,46.02 13.65,46.65 v25.72,46.65 | v25.72,53.95 OK101.4
CAN-L  (via drill 0.5)
  Top 0.61: v23.18,13.32 IC105.6 | v11.75,15.54 v11.75,35.54
  Bottom 0.61: X101.7 7.62,14.9 8.26,15.54 v11.75,15.54 13.02,15.54 13.34,15.86 18.1,15.86 20.64,13.32 v23.18,13.32 | X102.7 7.62,35.22 7.94,35.54 v11.75,35.54 11.75,47.29 12.7,48.24 R108.2
GND  (via drill 0.5)
  Top 0.406: 52.39,92.06 C104.-
  Top 0.61: IC103.4 47.94,10.46 48.58,9.82 61.28,9.82
  Top 0.813: IC101.31 C101.2 | C104.- 50.67,90.47 R107.2 44.77,85.39 | 44.77,85.39 44.77,85.07 43.81,84.12 IC102.1 | 24.77,86.66 V101.GND | 24.77,86.66 28.26,86.66 30.8,84.12 C106.2 IC102.1 | D101.K 11.43,77.13 20.95,86.66 24.77,86.66 | 61.28,93.64 OK201.9 | 61.28,88.56 61.28,93.64 | 61.28,83.48 61.28,88.56 | 61.28,78.4 61.28,83.48 | 61.28,72.37 61.28,78.4 | 61.28,66.97 61.28,72.37 | 61.28,62.21 61.28,66.97 | 61.28,57.13 61.28,62.21 | 61.28,51.1 61.28,57.13 | 61.28,51.1 61.28,46.02 | 61.28,46.02 61.28,40.94 | 61.28,40.94 61.28,35.86 | 61.28,24.75 61.28,19.66 | 61.28,19.66 61.28,14.59 | 61.28,14.59 OK204.15 | 61.28,19.66 OK204.13 | 61.28,24.75 OK204.11 | 61.28,29.82 OK204.9 | 61.28,29.82 61.28,24.75 | 61.28,35.86 OK203.15 | 61.28,35.86 61.28,29.82 | 61.28,40.94 OK203.13 | 61.28,46.02 OK203.11 | OK203.9 61.28,51.1 | 61.28,88.56 OK201.11 | 61.28,83.48 OK201.13 | 61.28,78.4 OK201.15 | 61.28,72.37 OK202.9 | OK202.11 60.96,67.29 61.28,66.97 | 61.28,62.21 OK202.13 | 61.28,57.13 OK202.15 | 61.28,93.64 v61.28,95.23 v60.01,95.23 v58.74,95.23 55.56,95.23 52.39,92.06 | C107.- 50.16,85.39 44.77,85.39 | 61.28,14.59 61.28,9.82 61.28,6.97 | 61.28,6.97 61.28,6.65 62.87,5.06 DC201.1 | SV101.6 29.53,6.33 28.26,7.6 IC105.8 28.26,11.09 25.72,13.63 IC105.2 25.72,18.08 26.35,18.71 32.07,18.71 32.7,19.35 IC104.9 29.53,23.16 24.45,28.24 QG101.7 | C105.2 36.83,80.94 38.1,82.21 IC102.1 | C202.2 61.28,6.97
  Top 1.27: v5.4,70.47 v9.21,70.47 17.14,62.53 17.14,59.99 | 17.14,59.99 v17.14,49.83 17.14,39.03 21.27,34.9 QG101.7 18.41,25.38 18.41,8.87 16.19,6.65 | C103.2 17.14,59.99 | X101.S@2 11.9,2.35 16.19,6.65 | 16.19,6.65 12.89,9.95 X101.4 X101.5 3.94,10.97 1.91,13 1.91,20.62 | X102.4 X102.3 7.62,30.14 | X102.4 X102.5 | X101.S@1 X102.S@2 8.51,20.68 8.57,20.62 1.91,20.62 | 1.91,30.14 7.62,30.14 | 7.62,30.14 9.21,30.14 X102.4 | X102.S@1 8.51,39.41 6.99,40.94 3.17,40.94 1.91,39.67 1.91,30.14 | 1.91,30.14 1.91,20.62
  Bottom 0.813: IC101.31 46.67,53.64 44.13,51.1 IC101.11 33.02,51.1 31.75,49.83 v17.14,49.83 12.06,49.83 8.57,46.33 8.57,38.4 | 73.98,42.21 IC202.2 | 73.98,42.21 IC202.3 | IC201.2 IC201.3 | IC201.2 IC201.1 73.98,71.42 73.03,72.37 73.03,94.59 72.39,95.23 v61.28,95.23 v60.01,95.23 v58.74,95.23 | 76.2,52.05 IC201.8 | 76.2,52.05 76.2,42.21 | 76.2,42.21 73.98,42.21 | IC201.2 75.56,67.29 76.2,66.66 76.2,52.05 | 52.39,51.1 OK203.9 | C101.2 52.39,51.1 | 76.2,42.21 76.2,28.87 75.56,28.24 IC202.8 73.98,26.33 73.03,25.38 73.03,8.87 72.07,7.92 69.22,7.92 68.26,6.97 DC201.1 | C102.2 52.39,51.1
  Bottom 1.27: 3.17,77.13 3.17,86.46 5.28,88.56 CON101.2 | 3.17,77.13 D101.K | 3.17,77.13 3.17,72.69 v5.4,70.47 v6.67,70.47 v7.94,70.47 v9.21,70.47
GNDA  (via drill 0.5)
  Top 2.184: 116.2,50.14 X203.1 | 116.2,50.14 X203.2 | v110.17,50.14 v108.9,50.14 | v110.17,50.14 v111.44,50.14 | v110.17,50.14 116.2,50.14
  Bottom 0.813: D216.A 85.41,4.74 81.92,8.24 81.92,13.95 81.28,14.59 C201.2 76.83,14.59 74.3,12.04 74.3,6.65 73.34,5.7 DC201.3
  Bottom 2.184: v110.17,50.14 v111.44,50.14 | v110.17,50.14 v108.9,50.14 | D216.A D215.A D214.A D213.A D212.A D211.A D210.A D209.A 88.58,50.14 | D201.A D202.A D203.A D204.A D205.A D206.A D207.A D208.A 88.58,50.14 | 88.58,50.14 v110.17,50.14
I00
  Top 0.406: IC101.35 50.16,63.8 50.8,64.43 50.8,80.31 54.93,84.44 54.93,89.52 56.52,91.1 OK201.10
I01
  Top 0.406: IC101.34 51.12,61.26 51.75,61.89 51.75,79.99 57.78,86.02 OK201.12
I02
  Top 0.406: IC101.33 51.75,58.72 52.7,59.67 52.7,79.67 53.98,80.94 OK201.14
I03  (via drill 0.5)
  Top 0.406: v40.32,67.61 v40.32,43.48
  Bottom 0.406: v40.32,43.48 IC101.14 | v40.32,67.61 53.98,67.61 54.61,68.24 54.61,73.96 56.52,75.86 OK201.16
I04  (via drill 0.5)
  Top 0.406: v41.27,65.07 v41.27,40.94
  Bottom 0.406: v41.27,40.94 IC101.15 | v41.27,65.07 54.93,65.07 55.56,65.7 55.56,68.88 56.52,69.83 OK202.10
I05  (via drill 0.5)
  Top 0.406: v42.23,62.53 v42.23,38.4
  Bottom 0.406: v42.23,38.4 IC101.16 | v42.23,62.53 54.93,62.53 57.15,64.75 OK202.12
I06  (via drill 0.5)
  Top 0.406: v43.18,59.99 v43.18,35.86
  Bottom 0.406: v43.18,35.86 IC101.17 | v43.18,59.99 57.15,59.99 57.47,59.67 OK202.14
I07  (via drill 0.5)
  Top 0.406: v46.35,33.32 46.35,51.41 47.31,52.37 54.29,52.37 56.52,54.59 OK202.16
  Bottom 0.406: v46.35,33.32 IC101.18
I08
  Top 0.406: IC101.29 49.53,48.56 51.44,46.65 54.93,46.65 56.83,48.56 OK203.10
I09
  Top 0.406: IC101.28 49.21,46.02 49.53,45.7 54.93,45.7 57.47,43.48 OK203.12
I10
  Top 0.406: IC101.26 51.75,40.94 54.29,38.4 OK203.14
I11
  Top 0.406: IC101.25 51.75,38.4 56.83,33.32 OK203.16
I12
  Top 0.406: IC101.24 52.39,35.86 53.66,34.59 53.66,28.87 55.24,27.29 OK204.10
I13
  Bottom 0.406: IC101.21 54.29,28.24 56.52,26.02 56.52,22.84 57.15,22.21 OK204.12
I14
  Bottom 0.406: IC101.19 43.18,30.78 46.99,26.97 54.29,26.97 55.56,25.7 55.56,18.71 57.15,17.12 OK204.14
I15
  Bottom 0.406: IC101.20 44.45,28.24 46.67,26.02 53.98,26.02 54.61,25.38 54.61,15.54 58.1,12.04 OK204.16
LED-G
  Top 0.406: IC101.2 32.7,74.28 R105.1
LED-R
  Bottom 0.61: IC101.4 32.38,68.88 R104.1
MISO  (via drill 0.5)
  Top 0.406: v39.37,61.26 39.37,32.05 46.67,24.75 46.67,20.93 45.4,19.66 IC104.15
  Bottom 0.406: SV101.1 43.5,8.87 45.4,10.78 IC104.15 45.4,17.12 46.04,17.76 51.12,17.76 51.75,17.12 51.75,13.63 53.02,12.36 IC103.2 | IC101.7 v39.37,61.26
MOSI  (via drill 0.5)
  Top 0.406: IC103.5 47.94,6.97 47.31,7.6 39.37,7.6 SV101.4 | IC104.14 42.86,19.66 44.13,20.93 44.13,24.75 38.42,30.46 v38.42,63.8
  Bottom 0.406: SV101.4 39.37,7.6 39.37,10.14 42.86,13.63 IC104.14 | v38.42,63.8 IC101.6
N$1  (via drill 0.5)
  Top 0.406: v32.38,13.32 29.84,13.32 28.26,14.9 IC105.1
  Bottom 0.406: IC104.1 53.02,21.25 52.07,20.3 38.73,20.3 36.51,18.08 36.51,13.95 35.88,13.32 v32.38,13.32
N$2  (via drill 0.5)
  Top 0.406: v29.21,12.04 v32.38,12.04 | v50.48,18.71 IC104.2
  Bottom 0.406: IC105.4 20.64,15.22 21.59,14.27 26.99,14.27 v29.21,12.04 | v32.38,12.04 37.15,12.04 39.05,13.95 39.05,18.08 39.69,18.71 v50.48,18.71
N$4
  Top 0.406: OK101.3 29.84,51.41 R108.1
N$6
  Bottom 0.813: C107.+ 44.77,87.93 33.34,87.93 | 33.34,87.93 D102.C 28.57,87.93 27.3,86.66 V101.IN | C106.1 33.34,87.93
N$7
  Top 0.406: R109.2 19.68,53.95 OK101.1
  Bottom 0.61: OK101.1 4.13,53.95 1.59,51.41 1.59,11.09 3.81,8.87 7.56,8.87 X101.3
N$9
  Bottom 0.406: D101.AR 8.57,74.59 11.75,71.42 R104.2
N$13
  Bottom 0.406: D101.AG 8.89,79.67 10.79,77.77 10.79,75.23 11.75,74.28 R105.2
N$15  (via drill 0.5)
  Top 0.406: IC201.9 84.77,52.05 85.72,51.1 93.03,51.1 v96.2,54.27
  Bottom 0.406: v96.2,54.27 97.16,55.22 106.05,55.22 107.31,53.95 108.9,53.95 109.54,54.59 LED203.K
N$16  (via drill 0.5)
  Top 0.406: RN204.6 83.19,17.12 84.14,16.17 84.14,14.59 85.09,13.63 v103.82,13.63
  Top 0.813: v103.82,13.63 114.62,13.63 116.2,12.04 X202.7
  Bottom 0.813: D215.C v103.82,13.63
N$17
  Top 0.406: RN204.8 72.71,12.04 73.34,12.68 73.34,15.54 73.98,16.17 82.55,16.17 83.19,15.54 83.19,9.19 83.82,8.55 94.61,8.55 98.42,4.74 D216.C
  Top 0.813: X202.8 116.2,7.28 114.94,8.55 107.63,8.55 D216.C
N$18
  Top 0.406: RN204.2 71.75,27.29 72.07,26.97 84.45,26.97 86.36,25.06 98.74,25.06 100.97,22.84 104.14,22.84
  Top 0.813: X202.5 116.2,22.52 114.94,23.79 107.63,23.79 106.68,22.84 104.14,22.84 D213.C
N$19  (via drill 0.5)
  Top 0.406: RN204.4 72.39,22.21 73.03,22.84 73.03,25.38 73.66,26.02 82.55,26.02 85.09,23.48 85.09,20.3 85.72,19.66 v103.82,19.66
  Top 0.813: v103.82,19.66 107.63,19.66 108.58,18.71 114.94,18.71 116.2,17.44 X202.6
  Bottom 0.813: D214.C v103.82,19.66
N$20
  Top 0.406: RN203.6 72.07,37.13 84.77,37.13 85.09,36.81 94.61,36.81 96.52,34.9 104.14,34.9
  Top 0.813: X202.3 116.2,32.68 114.94,33.95 107.63,33.95 106.68,34.9 104.14,34.9 D211.C
N$21
  Top 0.406: RN203.8 72.07,32.05 83.82,32.05 85.09,30.78 94.61,30.78 96.52,28.87 105.09,28.87
  Top 0.813: X202.4 116.2,27.6 114.94,28.87 105.09,28.87 D212.C
N$22
  Top 0.406: RN203.2 100.33,48.56 101.92,46.97 D209.C
  Top 0.813: X202.1 115.25,42.52 115.25,45.06 114.62,45.7 110.81,45.7 109.54,46.97 D209.C
N$23
  Top 0.406: RN203.4 72.07,42.21 83.19,42.21 86.36,39.03 97.79,39.03 99.69,40.94 D210.C
  Top 0.813: X202.2 116.2,37.76 114.94,39.03 108.58,39.03 106.68,40.94 D210.C
N$24
  Top 0.406: RN202.6 70.8,59.99 71.75,60.94 85.09,60.94 85.41,61.26 97.47,61.26 99.69,59.03 D207.C
  Top 0.813: X201.7 115.89,63.48 113.35,63.48 111.12,61.26 108.9,61.26 106.36,59.03 D207.C
N$25
  Top 0.406: RN202.8 72.07,55.86 84.14,55.86 84.45,56.18 110.49,56.18 110.49,55.86
  Top 0.813: X201.8 113.35,58.72 110.49,55.86 110.49,54.59 108.9,53 D208.C
N$26
  Top 0.406: RN202.2 71.44,69.83 73.03,71.42 84.45,71.42 85.72,72.69 99.06,72.69 100.65,71.1 D205.C
  Top 0.813: D205.C 106.36,71.1 106.68,71.42 110.49,71.42 113.03,73.96 X201.5
N$27
  Top 0.406: RN202.4 70.8,65.07 71.75,66.02 84.14,66.02 85.41,67.29 96.2,67.29 98.42,65.07 D206.C
  Top 0.813: D206.C 106.36,65.07 107.63,66.34 112.71,66.34 115.25,68.88 X201.6
N$28
  Top 0.406: RN201.6 72.39,80.94 74.3,82.85 82.23,82.85 83.82,81.26 96.84,81.26 98.74,83.17 D203.C
  Top 0.813: X201.3 113.35,84.12 110.81,81.58 108.58,81.58 107,83.17 D203.C
N$29
  Top 0.406: RN201.8 72.71,75.86 74.93,73.64 82.55,73.64 83.82,74.91 94.3,74.91 96.52,77.13 D204.C
  Top 0.813: X201.4 113.03,79.04 110.49,76.5 107.31,76.5 106.68,77.13 106.36,77.13 D204.C
N$30
  Top 0.406: RN201.2 75.88,91.1 77.47,92.69 103.5,92.69 103.82,92.37 104.78,91.74
  Top 0.813: X201.1 113.35,94.28 110.81,91.74 104.78,91.74 104.46,91.74 103.82,92.37 D201.C
N$31  (via drill 0.5)
  Top 0.406: v108.27,55.22 85.09,55.22 84.45,54.59 IC201.10
  Bottom 0.406: v108.27,55.22 108.27,61.26 LED211.K
N$32
  Top 0.406: OK204.2 RN204.7
N$35
  Top 0.406: OK204.4 RN204.5
N$36
  Top 0.406: OK204.6 RN204.3
N$37
  Top 0.406: OK204.8 RN204.1
N$38
  Top 0.406: OK203.2 RN203.7
N$39
  Top 0.406: OK203.4 RN203.5
N$40
  Top 0.406: OK203.6 RN203.3
N$41
  Top 0.406: OK203.8 RN203.1
N$42
  Top 0.406: OK202.2 RN202.7
N$43
  Top 0.406: OK202.4 RN202.5
N$44
  Top 0.406: OK202.6 RN202.3
N$45
  Top 0.406: OK202.8 RN202.1
N$46
  Top 0.406: OK201.2 RN201.7
N$47
  Top 0.406: RN201.4 96.84,86.02 100.01,89.2 D202.C
  Top 0.813: X201.2 113.35,89.2 110.81,86.66 104.78,86.66 103.82,87.61 D202.C
N$48
  Top 0.406: OK201.4 RN201.5
N$49  (via drill 0.5)
  Top 0.406: v86.04,42.84 107,42.84 LED205.K | v78.42,39.67 77.47,39.67 76.2,38.4 IC202.4
  Bottom 0.406: v86.04,42.84 82.87,39.67 v78.42,39.67
N$50  (via drill 0.5)
  Top 0.406: v69.22,73.96 73.34,73.96 v74.61,72.69 | v85.09,91.1 v101.6,91.1
  Bottom 0.406: IC201.4 73.98,61.89 73.03,60.94 65.72,60.94 65.09,61.57 65.09,73.32 65.72,73.96 v69.22,73.96 | v74.61,72.69 78.11,72.69 81.6,76.18 81.6,87.61 v85.09,91.1 | v101.6,91.1 103.5,93.01 LED201.K
N$51  (via drill 0.5)
  Top 0.406: v77.47,59.67 IC201.5 | v92.71,86.98 v82.87,86.98
  Bottom 0.406: v77.47,59.67 77.47,70.78 82.87,76.18 v82.87,86.98 | LED209.K 107.31,87.93 106.36,86.98 v92.71,86.98
N$52  (via drill 0.5)
  Top 0.406: v78.42,57.13 IC201.6 | LED202.K 107.31,85.07 v84.14,85.07
  Bottom 0.406: v78.42,57.13 78.42,70.47 84.14,76.18 v84.14,85.07
N$53  (via drill 0.5)
  Top 0.406: v79.38,54.59 IC201.7 | LED210.K 107.95,79.36 v85.41,79.36
  Bottom 0.406: v79.38,54.59 79.38,70.15 80.96,71.73 85.41,75.86 v85.41,79.36
N$54  (via drill 0.5)
  Top 0.406: v107.31,57.13 IC201.11
  Bottom 0.406: v107.31,57.13 107.31,65.39 LED204.K
N$55  (via drill 0.5)
  Top 0.406: v84.77,59.67 IC201.12 | LED212.K 108.58,73.64 v84.77,73.64
  Bottom 0.406: v84.77,73.64 v84.77,59.67
N$56  (via drill 0.5)
  Top 0.406: v84.77,7.6 93.66,7.6 98.74,2.52 107.31,2.52 LED207.K
  Bottom 0.406: IC202.9 82.55,28.24 83.19,27.6 83.19,9.19 v84.77,7.6
N$57  (via drill 0.5)
  Top 0.406: LED213.K 107,37.76 85.41,37.76 85.09,38.08 83.5,39.67 80.01,39.67 78.74,38.4 v78.42,38.4 | IC202.5 v78.42,35.86
  Bottom 0.406: v78.42,35.86 v78.42,38.4
N$58
  Top 0.406: LED206.K 107.95,31.73 85.72,31.73 82.87,34.59 77.47,34.59 76.2,33.32 IC202.6
N$59
  Top 0.406: LED214.K 108.27,26.33 86.68,26.33 85.72,27.29 83.5,29.51 77.47,29.51 76.2,30.78 IC202.7
N$60  (via drill 0.5)
  Top 0.406: v85.09,12.68 106.68,12.68 LED215.K
  Bottom 0.406: IC202.10 83.19,30.78 84.14,29.82 84.14,13.63 v85.09,12.68
N$61  (via drill 0.5)
  Top 0.406: v86.36,18.71 106.68,18.71 107.95,17.44 107.95,15.86 108.9,14.9 LED208.K
  Bottom 0.406: IC202.11 84.14,33.32 85.09,32.36 85.09,19.98 v86.36,18.71
N$62  (via drill 0.5)
  Top 0.406: IC202.12 83.82,35.86 87,32.68 v97.16,32.68 | v97.16,22.21 98.42,20.93 108.58,20.93 LED216.K
  Bottom 0.406: v97.16,32.68 v97.16,22.21
N$64
  Top 0.406: OK201.6 RN201.3
N$65
  Top 0.406: OK201.8 RN201.1
PLUGGED  (via drill 0.5)
  Top 0.406: v13.34,76.5 v13.34,73.01 | v40.01,73.96 IC101.39
  Bottom 0.406: CON101.3 10.65,79.18 v13.34,76.5 | v13.34,73.01 31.11,73.01 31.43,72.69 38.73,72.69 v40.01,73.96
Q-CLK
  Top 0.61: IC101.13 33.02,46.02 30.8,43.79 30.8,28.24 | 30.8,28.24 QG101.8 | 30.8,28.24 30.8,27.6 32.38,26.02 34.29,26.02 35.24,25.06 IC104.8
SCK  (via drill 0.5)
  Top 0.406: IC103.6 50.48,7.6 49.21,8.87 45.72,8.87 44.13,10.46 38.42,10.46 38.1,10.14 SV101.3 | IC104.13 40.32,19.66 41.59,20.93 41.59,24.75 37.47,28.87 v37.47,58.72
  Bottom 0.406: SV101.3 38.1,11.09 40.32,13.32 IC104.13 | v37.47,58.72 IC101.8
SCL  (via drill 0.5)
  Top 0.406: IC201.14 83.19,64.75 85.09,62.84 107.31,62.84 108.27,63.8 v111.76,63.8 | v111.76,52.37 111.44,52.05 107.31,52.05 105.41,50.14 v86.04,50.14 | v78.74,47.29 v72.39,47.29
  Bottom 0.406: IC101.22 52.39,30.78 53.66,29.51 R201.1 56.2,28.55 64.45,28.55 65.09,29.19 65.09,46.65 65.72,47.29 v72.39,47.29 | v111.76,63.8 v111.76,52.37 | v86.04,50.14 85.41,49.51 85.41,43.79 82.55,40.94 IC202.14 79.69,40.94 78.74,41.89 v78.74,47.29
SDA  (via drill 0.5)
  Top 0.406: v79.69,49.83 v72.39,49.83
  Bottom 0.406: IC101.23 R202.1 53.66,31.73 62.87,31.73 64.14,33 64.14,48.24 65.72,49.83 v72.39,49.83 | IC201.15 83.5,67.29 83.82,66.97 83.82,43.79 83.5,43.48 IC202.15 80.64,43.48 79.69,44.43 v79.69,49.83
SPG
  Bottom 0.61: R106.2 R107.1 44.77,78.72 46.99,76.5 IC101.40
V+
  Top 0.813: OK201.7 65.72,91.1 65.09,90.47 65.09,86.02 | 65.09,86.02 65.09,80.94 | 65.09,80.94 65.09,75.86 | 65.09,75.86 65.09,69.83 | 65.09,69.83 65.09,64.75 | 65.09,64.75 65.09,59.67 | 65.09,59.67 65.09,54.59 | 65.09,54.59 65.09,48.56 | 65.09,48.56 65.09,43.48 | 65.09,43.48 65.09,38.08 | 65.09,38.08 65.09,33.32 | 65.09,33.32 65.09,27.29 | 65.09,27.29 65.09,22.21 | 65.09,22.21 65.09,16.81 | 65.09,16.81 65.09,12.04 | 65.09,12.04 65.09,9.82 65.72,9.19 74.3,9.19 75.88,7.6 DC201.4 | 65.09,12.04 OK204.1 | OK204.3 65.41,17.12 65.09,16.81 | 65.09,22.21 OK204.5 | 65.09,27.29 OK204.7 | OK203.3 65.41,38.4 65.09,38.08 | 65.09,43.48 OK203.5 | 65.09,48.56 OK203.7 | 65.09,59.67 OK202.3 | 65.09,64.75 OK202.5 | 65.09,69.83 OK202.7 | 65.09,75.86 OK201.1 | 65.09,80.94 OK201.3 | 65.09,86.02 OK201.5 | 65.09,54.59 OK202.1 | 65.09,33.32 OK203.1
  Bottom 0.813: C201.1 76.83,12.04 75.88,11.09 DC201.4
V-NETZTEIL1
  Bottom 1.27: CON101.1 19.05,90.47 21.91,93.33 D103.A

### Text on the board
Bottom: MBCAN-Projekt | (c) Dr.-Ing. Th. Wiesner | 20.10.2022 | mbc88.brd | bottom
tNames: HW: 23.11.25 | 1 | 2 | +18V | DC | 3 | Status | 4 | 5 | 6 | (c) Dr.-Ing. Th. Wiesner | MBCAN-Projekt | 7 | 8 | 9 | IN | 10 | 11 | 12 | 13 | OUT | 14 | 15 | 16 | mbc-90-AC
